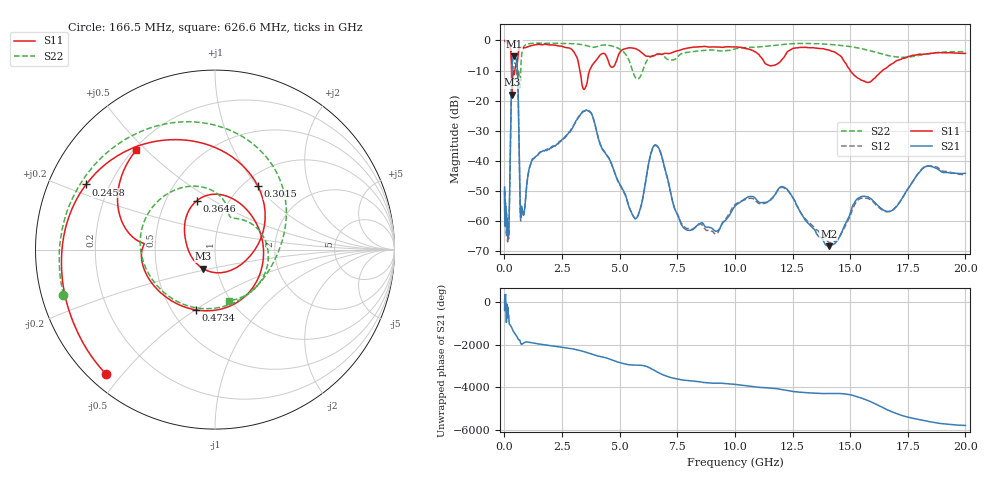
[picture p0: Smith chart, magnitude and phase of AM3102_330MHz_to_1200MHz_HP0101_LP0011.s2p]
! Date/Time: Tue, Sep 11, 2018 5:13 PM
! Network Analyzer: Agilent Technologies E8362B Rev: A.07.50.63
! Sweep from 0.010 to 20.000 GHz, 1601 Points, Sweep Type: LOG
! Power Supply: 4.949 V, 0.001 A
# Hz S DB R 50
!freq MagS11 AngS11 MagS21 AngS21 MagS12 AngS12 MagS22 AngS22
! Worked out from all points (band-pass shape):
!   1601 points, 10 MHz to 20 GHz, reference 50 ohm
!   highest |S21| = -5.27 dB at 420.4 MHz (marker M1); lowest = -68.3 dB at 14.07 GHz (marker M2)
!   |S21| within 3 dB of the highest: 335.6 MHz to 552.8 MHz (217.2 MHz wide, 48.9 % of centre)
!   lowest |S11| = -18.0 dB at 333.1 MHz (marker M3), VSWR 1.29, Z = 42.8 - j9.21 ohm
!   |S11| at or under -10 dB: 309.5 MHz to 450.3 MHz (140.7 MHz wide, 37 % of centre); 3.28 GHz to 3.694 GHz (413.9 MHz wide, 11.9 % of centre); 15.01 GHz to 16.4 GHz (1.399 GHz wide, 8.9 % of centre)
!   |S22| runs from -15.9 to -0.2 dB; largest |S21 - S12| = 0.0082
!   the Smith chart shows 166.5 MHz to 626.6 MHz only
!   S11 on the Smith chart (normalised r, x): 166.5 MHz: 0.05, -0.45; 245.8 MHz: 0.11, +0.24; 301.5 MHz: 1.16, +1.00; 364.6 MHz: 0.71, +0.43; 473.4 MHz: 0.66, -0.50; 626.6 MHz: 0.21, +0.47
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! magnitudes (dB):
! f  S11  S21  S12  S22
! 10 MHz  0.0  -48.7  -49.9  -0.2
! 35.55 MHz  0.0  -57.7  -60.6  -0.4
! 126.4 MHz  -0.4  -62.5  -62.1  -0.9
! 166.5 MHz  -0.7  -62.6  -63.5  -1.1
! 245.8 MHz  -1.9  -42.9  -43.0  -2.0
! 301.5 MHz  -7.4  -17.2  -17.3  -4.5
! 333.1 MHz  -18.0  -8.6  -8.7  -8.8
! 364.6 MHz  -10.7  -6.2  -6.3  -10.1
! 420.4 MHz  -11.4  -5.3  -5.3  -8.1
! 447.2 MHz  -10.1  -5.4  -5.4  -7.5
! 473.4 MHz  -9.1  -5.6  -5.7  -7.5
! 561.8 MHz  -7.6  -9.3  -9.4  -14.0
! 626.6 MHz  -3.0  -29.4  -29.4  -10.6
! 709 MHz  -2.3  -59.0  -60.0  -10.1
! 1.59 GHz  -1.4  -37.0  -37.0  -0.9
! 3.651 GHz  -11.1  -23.4  -23.2  -1.9
! 5.652 GHz  -2.6  -59.1  -59.0  -11.9
! 6.58 GHz  -4.7  -34.7  -34.9  -4.8
! 7.882 GHz  -2.7  -62.9  -62.3  -4.0
! 12.09 GHz  -6.0  -48.6  -48.8  -1.3
! 14.07 GHz  -3.2  -68.3  -67.0  -1.3
! 20 GHz  -4.3  -44.1  -44.7  -3.7
